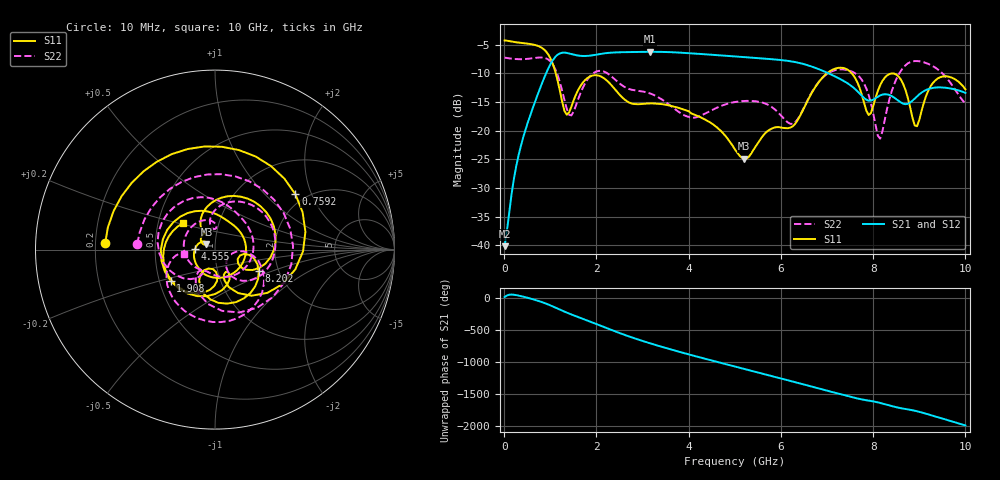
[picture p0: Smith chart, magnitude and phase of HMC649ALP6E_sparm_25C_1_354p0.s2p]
!Analog Devices Inc..
!GaAs MMIC 6-BIT DIGITAL PHASE SHIFTER, 3 - 6 GHz
!Filename: HMC649ALP6E_sparm_25C_1_354p0.s2p
!  :25C = 25degC
!  :_1_ = Sn1
!  :_354p0  = 354.0 state
!Device type:
!2 Port Calibration to sma connectors
!Phase Shifter:  0.000
!	Vss= -5V, Vdd= +5V , control Voltage = 0/ +5V
!Freq	S11	S11	S21	S21	S12	S12	S22	S22
! GHz	Mag dB	Degrees	Mag dB	Degrees	Mag dB	Degrees	Mag dB	Degrees
# GHZ S DB R 50.0
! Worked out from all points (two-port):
!   201 points, 10 MHz to 10 GHz, reference 50 ohm
!   highest |S21| = -6.24 dB at 3.157 GHz (marker M1); lowest = -40.1 dB at 10 MHz (marker M2)
!   |S21| within 3 dB of the highest: 952 MHz to 6.812 GHz (5.86 GHz wide, 151 % of centre)
!   lowest |S11| = -24.9 dB at 5.205 GHz (marker M3), VSWR 1.12, Z = 45.4 + j2.88 ohm
!   |S11| at or under -10 dB: 1.119 GHz to 6.999 GHz (5.879 GHz wide, 145 % of centre); 7.537 GHz to end of sweep
!   |S22| runs from -21.4 to -7.2 dB; largest |S21 - S12| = 0.0012
!   S11 on the Smith chart (normalised r, x): 10 MHz: 0.24, +0.03; 759.2 MHz: 1.76, +1.54; 1.908 GHz: 0.57, -0.22; 4.555 GHz: 0.80, +0.01; 8.202 GHz: 1.58, -0.41; 10 GHz: 0.67, +0.21
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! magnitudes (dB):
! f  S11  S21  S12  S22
! 10 MHz  -4.3  -40.1  -39.5  -7.2
! 309.7 MHz  -4.6  -24.4  -24.4  -7.5
! 759.2 MHz  -5.3  -13.0  -13.0  -7.2
! 1.059 GHz  -8.4  -7.7  -7.6  -8.5
! 1.359 GHz  -17.2  -6.4  -6.4  -16.2
! 1.708 GHz  -11.6  -7.0  -7.0  -12.5
! 1.908 GHz  -10.4  -6.9  -6.8  -10.1
! 3.157 GHz  -15.2  -6.2  -6.2  -13.5
! 3.357 GHz  -15.3  -6.2  -6.2  -14.2
! 4.555 GHz  -19.1  -6.8  -6.8  -16.2
! 5.005 GHz  -23.3  -7.0  -7.0  -15.0
! 5.205 GHz  -24.9  -7.2  -7.2  -14.8
! 6.254 GHz  -19.2  -7.9  -7.9  -18.8
! 6.703 GHz  -12.9  -8.9  -8.9  -12.8
! 7.602 GHz  -10.7  -12.7  -12.7  -9.9
! 7.902 GHz  -17.3  -14.8  -14.8  -13.8
! 8.102 GHz  -13.0  -14.1  -14.1  -20.9
! 8.202 GHz  -11.3  -13.7  -13.7  -20.1
! 8.352 GHz  -10.1  -13.8  -13.8  -14.5
! 8.951 GHz  -19.2  -14.0  -14.0  -7.9
! 9.401 GHz  -10.9  -12.4  -12.4  -9.3
! 10 GHz  -12.8  -13.4  -13.4  -15.2
